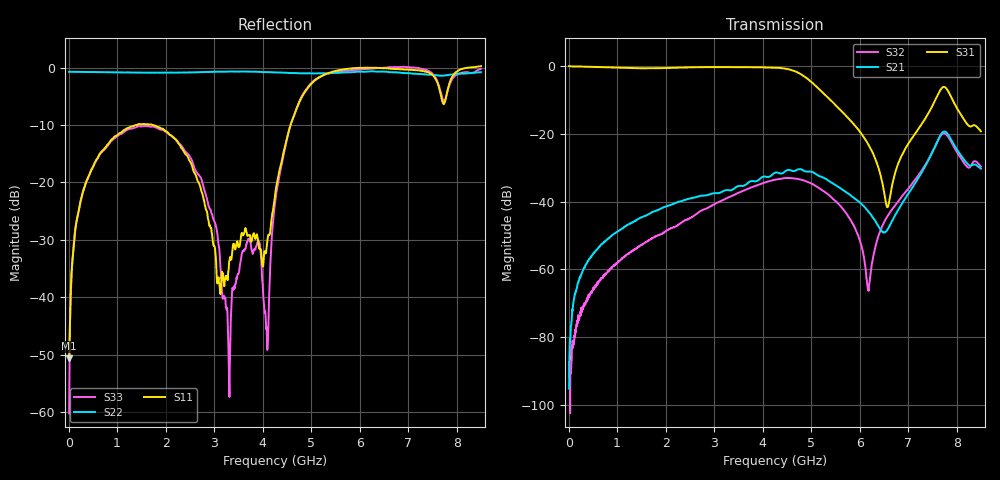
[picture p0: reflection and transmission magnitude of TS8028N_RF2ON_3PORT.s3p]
!Created with skrf (http://scikit-rf.org).
# GHz S RI R 50.0
!freq ReS11 ImS11 ReS12 ImS12 ReS13 ImS13
! ReS21 ImS21 ReS22 ImS22 ReS23 ImS23
! ReS31 ImS31 ReS32 ImS32 ReS33 ImS33
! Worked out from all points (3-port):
!   1601 points, 10 MHz to 8.5 GHz, reference 50 ohm
!   strongest paths, dB at 10 MHz, 2.132 GHz, 4.255 GHz, 6.378 GHz, 8.5 GHz:
!     S31: 0.0, -0.5, -0.5, -29.6, -19.3
!     S21: -95.2, -40.8, -31.5, -47.0, -30.3
!     S32: -87.4, -47.8, -33.5, -50.6, -29.6
!   lowest |S11| = -50.7 dB at 10 MHz (marker M1), VSWR 1.01, Z = 50.3 + j0.0406 ohm
!   |S11| at or under -10 dB: start of sweep to 1.406 GHz; 1.74 GHz to 4.576 GHz (2.836 GHz wide, 89.8 % of centre)
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0.01  0.00291 0.000403  3.02e-05 3.68e-05  0.9946 -0.00926
      -8.77e-06 1.5e-05  -0.9194 0.00506  -3.27e-06 1.67e-05
      0.9946 -0.00935  3.2e-05 2.82e-05  0.000456 0.000861
0.1851062  0.0027 -0.0505  -1.41e-05 0.00061  0.9791 -0.0941
           -7.08e-06 0.000614  -0.9168 0.0552  -5.71e-05 -0.000148
           0.979 -0.094  -6.21e-05 -0.000148  0.00228 -0.0515
0.9439  -0.102 -0.228  -0.000282 0.00337  0.8476 -0.4225
        -0.000288 0.00337  -0.8759 0.255  -0.00113 -0.000224
        0.8474 -0.4226  -0.00111 -0.000208  -0.1093 -0.216
2.51455  -0.1212 -0.0872  0.00221 0.011  0.361 -0.8852
         0.00223 0.0109  -0.6675 0.6159  -0.00459 0.00341
         0.3611 -0.8852  -0.00461 0.00343  -0.1455 -0.076
3.305181  0.0191 0.00145  0.00479 0.0139  -0.0926 -0.959
          0.00481 0.0139  -0.522 0.7627  -0.00524 0.0104
          -0.0926 -0.9592  -0.00522 0.0104  -0.00133 0.00153
4.255  -0.0456 0.0621  0.016 0.0214  -0.7287 -0.6047
       0.016 0.0213  -0.3538 0.8371  0.0083 0.0193
       -0.7291 -0.604  0.00827 0.0194  -0.00796 0.065
6.175863  0.754 0.6541  0.00706 -0.00139  -0.0399 0.0582
          0.00707 -0.00136  0.1425 0.9118  0.00041 0.00029
          -0.0397 0.0582  0.000401 0.000288  0.9447 0.2365
6.579137  0.7861 0.5918  0.00157 0.00356  -0.00734 -0.00393
          0.00162 0.00358  0.1855 0.8984  -0.00269 0.00553
          -0.00731 -0.00391  -0.00265 0.00557  0.9954 0.1353
7.688144  0.4451 0.308  0.0533 0.0859  -0.2871 -0.3699
          0.0531 0.0858  0.4597 0.7153  0.066 0.071
          -0.2857 -0.3697  0.0663 0.071  0.571 0.0595
8.5  0.4864 0.9075  0.0259 -0.0165  -0.0845 0.0685
     0.0258 -0.0165  0.6201 0.6694  0.0204 -0.026
     -0.0846 0.0687  0.0204 -0.0259  0.855 0.4694
